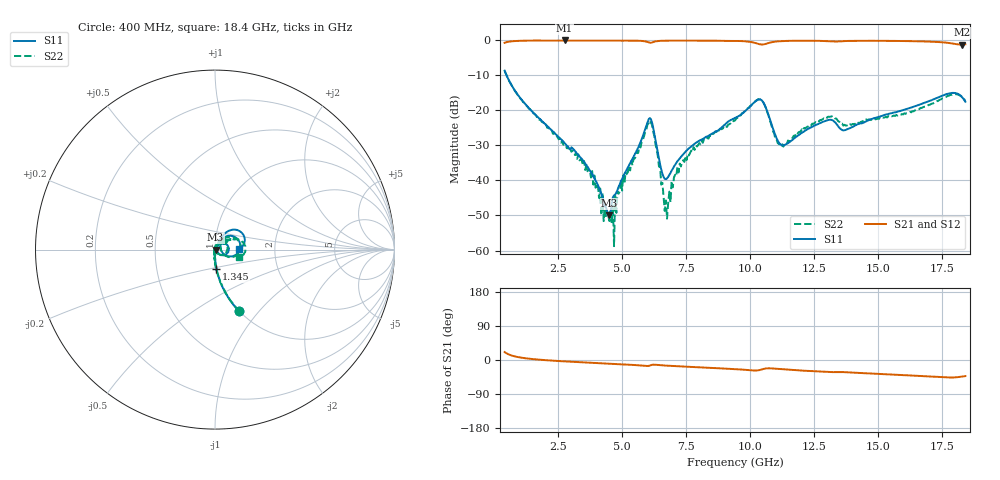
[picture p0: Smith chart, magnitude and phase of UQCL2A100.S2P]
! AVX Corporation
! Date:  10/27/06
! Part No:  UQCL2A100
! Description:  Ultra Low ESR Microwave capacitors
! Mounting Orientation:  Horizontal
# GHZ S DB R 50
! Freq  |S11|  S11 Ph  |S21|  S21 Ph  |S12|  S12 Ph  |S22|  S22 Ph
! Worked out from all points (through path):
!   401 points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, 400 MHz to 18.4 GHz, reference 50 ohm
!   highest |S21| = -0.01 dB at 2.74 GHz (marker M1); lowest = -1.2 dB at 18.27 GHz (marker M2)
!   group delay of S21, straight-line fit = 7.88 ps
!   lowest |S11| = -50.0 dB at 4.495 GHz (marker M3), VSWR 1.01, Z = 50.3 - j0.0276 ohm
!   |S11| at or under -10 dB: 478.3 MHz to end of sweep
!   |S22| runs from -58.8 to -8.6 dB; largest |S21 - S12| = 0.0017
!   S11 on the Smith chart (normalised r, x): 400 MHz: 1.00, -0.79; 1.345 GHz: 0.99, -0.22; 18.4 GHz: 1.31, +0.02
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0.4  -8.64 -68.5  -0.68 20.9  -0.68 21.0  -8.62 -68.4
1.345  -19.30 -85.8  -0.06 3.5  -0.06 3.5  -19.45 -87.1
2.74  -29.29 -91.4  -0.01 -3.6  -0.02 -3.6  -29.65 -94.5
3.415  -33.83 -89.4  -0.02 -6.2  -0.02 -6.1  -34.29 -92.6
4.495  -49.96 -5.0  -0.03 -9.7  -0.03 -9.7  -51.60 104.2
4.675  -44.25 24.4  -0.02 -10.3  -0.02 -10.3  -58.76 94.3
4.945  -40.20 47.0  -0.03 -11.2  -0.03 -11.2  -40.31 101.6
6.025  -22.54 17.6  -0.55 -15.5  -0.55 -15.5  -23.67 22.9
6.16  -23.48 -24.0  -0.59 -12.8  -0.58 -12.7  -24.10 -23.6
6.43  -33.82 -44.8  -0.15 -13.4  -0.14 -13.3  -36.01 -64.8
6.7  -39.64 5.0  -0.07 -14.8  -0.07 -14.7  -45.69 -2.4
7.15  -34.51 50.3  -0.05 -16.5  -0.05 -16.5  -36.18 70.7
7.465  -31.80 56.8  -0.05 -17.5  -0.05 -17.5  -33.02 68.0
9.4  -22.13 55.3  -0.15 -23.9  -0.15 -23.9  -22.88 51.1
10.39  -16.87 7.5  -1.13 -26.1  -1.13 -26.1  -16.79 3.6
11.245  -30.03 7.1  -0.20 -24.4  -0.19 -24.4  -29.65 12.9
12.415  -24.69 48.8  -0.10 -29.5  -0.09 -29.5  -23.77 50.7
13.135  -22.66 39.3  -0.25 -32.0  -0.25 -31.9  -21.77 39.2
13.675  -25.66 45.1  -0.19 -32.1  -0.19 -32.0  -24.10 34.8
15.43  -20.90 59.9  -0.13 -38.1  -0.13 -38.0  -21.85 39.0
18.265  -16.18 7.4  -1.18 -43.7  -1.19 -43.7  -16.14 -11.5
18.4  -17.51 2.5  -1.09 -42.5  -1.09 -42.4  -17.25 -17.2
